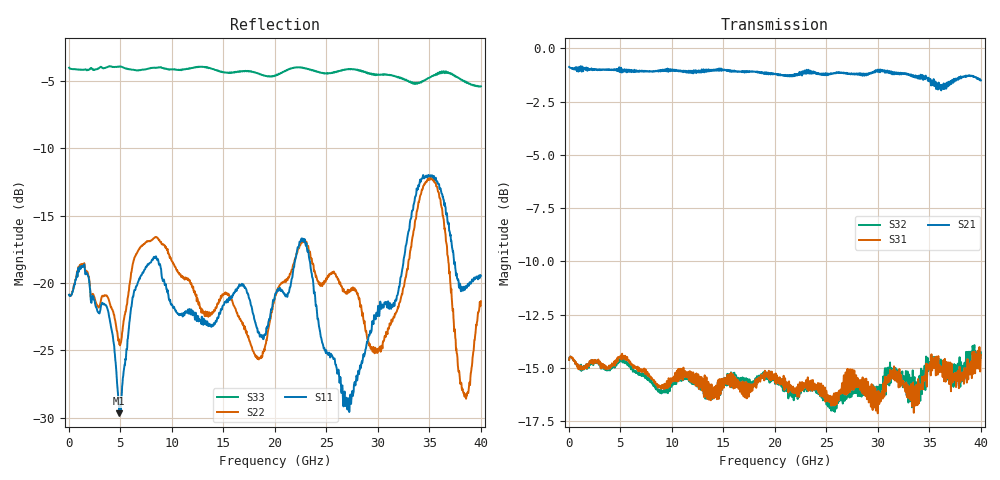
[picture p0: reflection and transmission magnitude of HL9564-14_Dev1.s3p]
! 1/20/2021 10:06:25 AM
! H:\PRODUCTION_DATA\TEMP_S3P.S3P
! CHANNEL.1
! TR.MEASUREMENT
! CORRECTED.DATA
# GHZ S RI R 50.0
! FREQ.GHZ  S11RE  S11IM  S12RE  S12IM  S13RE  S13IM
!  S21RE  S21IM  S22RE  S22IM  S23RE  S23IM
!  S31RE  S31IM  S32RE  S32IM  S33RE  S33IM
!; PortSelection: Port_123
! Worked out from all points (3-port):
!   1143 points, 35 MHz to 40.01 GHz, reference 50 ohm
!   strongest paths, dB at 35 MHz, 10.01 GHz, 20.02 GHz, 30.03 GHz, 40.01 GHz:
!     S21: -0.9, -1.1, -1.2, -1.1, -1.5
!     S31: -14.6, -15.5, -15.7, -16.5, -14.4
!     S32: -14.6, -15.7, -15.7, -15.9, -14.3
!   lowest |S11| = -29.7 dB at 4.9 GHz (marker M1), VSWR 1.07, Z = 46.8 + j0.292 ohm
!   |S11| at or under -10 dB: start of sweep to end of sweep
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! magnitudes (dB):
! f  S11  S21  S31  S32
! 35 MHz  -20.9  -0.9  -14.6  -14.6
! 4.9 GHz  -29.7  -0.9  -14.5  -14.7
! 8.295 GHz  -18.1  -1.1  -15.7  -15.8
! 20.02 GHz  -20.9  -1.2  -15.7  -15.7
! 22.89 GHz  -16.7  -1.0  -15.9  -15.8
! 27.09 GHz  -28.8  -1.2  -15.7  -16.3
! 30.27 GHz  -21.6  -1.0  -16.6  -16.4
! 35.14 GHz  -12.0  -1.6  -15.3  -15.0
! 38.33 GHz  -20.4  -1.3  -15.2  -15.3
! 40.01 GHz  -19.5  -1.5  -14.4  -14.3
